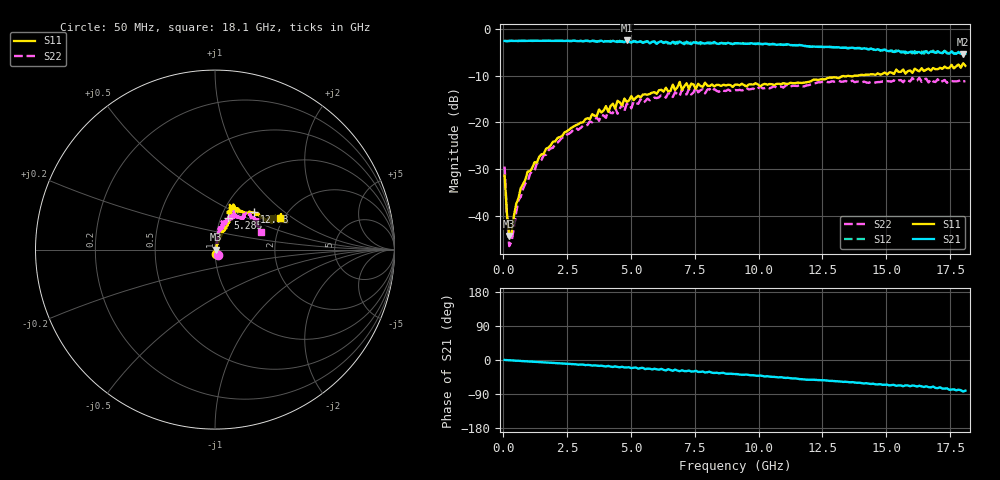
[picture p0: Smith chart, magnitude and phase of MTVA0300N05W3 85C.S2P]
! Network Analyzer HP8720D.06.14 Serial No. US36140669
!  7 Jul 2005  09:27:54
! Frequency  S11  S21  S12  S22
# HZ  S  DB R 50
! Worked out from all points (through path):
!   201 points, 50 MHz to 18.1 GHz, reference 50 ohm
!   highest |S21| = -2.42 dB at 4.833 GHz (marker M1); lowest = -5.3 dB at 18.01 GHz (marker M2)
!   group delay of S21, straight-line fit = 12.3 ps
!   lowest |S11| = -44.4 dB at 230.5 MHz (marker M3), VSWR 1.01, Z = 50.6 - j0.127 ohm
!   |S11| at or under -10 dB: start of sweep to 13.74 GHz; 13.83626 GHz to 13.87192 GHz (35.66 MHz wide, 0.257 % of centre)
!   |S22| runs from -46.6 to -10.4 dB; largest |S21 - S12| = 0.045
!   S11 on the Smith chart (normalised r, x): 50 MHz: 1.02, -0.05; 5.285 GHz: 1.08, +0.40; 12.78 GHz: 1.39, +0.64; 18.1 GHz: 1.93, +0.80
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5e7  -31.42 -72.1  -2.52 0.1  -2.51 0.2  -29.48 -61.3
1.4025e8  -39.49 -54.7  -2.56 -0.4  -2.56 -0.4  -39.91 -62.7
2.305e8  -44.39 -12.0  -2.53 -0.7  -2.52 -0.8  -46.57 -31.9
3.2075e8  -43.78 33.0  -2.50 -0.9  -2.52 -1.0  -45.61 32.0
5.915e8  -36.28 63.3  -2.52 -2.0  -2.54 -2.1  -36.69 71.9
1.04275e9  -30.49 70.9  -2.48 -4.0  -2.50 -4.0  -31.09 73.4
1.94525e9  -24.15 68.6  -2.51 -7.8  -2.51 -7.7  -25.44 77.1
3.1185e9  -20.01 67.6  -2.58 -12.0  -2.60 -12.5  -20.72 78.9
4.83325e9  -15.60 71.0  -2.42 -19.5  -2.69 -20.3  -16.07 67.5
5.2845e9  -14.29 67.8  -2.76 -23.0  -2.83 -22.2  -16.04 67.0
6.09675e9  -13.11 65.0  -2.77 -25.6  -2.66 -25.2  -14.62 66.7
6.7285e9  -13.08 71.6  -2.85 -25.4  -3.17 -26.5  -13.53 60.8
6.909e9  -11.32 67.8  -2.65 -29.6  -2.77 -27.4  -14.32 61.1
6.99925e9  -13.02 67.7  -2.97 -27.3  -3.15 -29.8  -12.92 61.4
7.17975e9  -11.61 71.8  -2.69 -29.3  -3.02 -27.6  -14.01 57.6
7.54075e9  -12.81 64.4  -2.94 -28.5  -2.79 -31.9  -12.44 64.1
9.075e9  -11.89 64.2  -3.03 -37.0  -2.99 -37.1  -13.06 54.8
1.21435e10  -10.85 47.7  -3.72 -52.1  -3.66 -52.1  -11.69 50.2
1.277525e10  -10.38 43.4  -3.80 -55.1  -3.82 -54.7  -11.38 45.7
1.512175e10  -9.26 27.1  -4.72 -67.1  -4.45 -66.6  -11.21 39.5
1.800975e10  -7.32 20.6  -5.32 -83.3  -5.03 -83.2  -11.26 25.4
1.81e10  -7.87 25.5  -5.24 -80.9  -5.54 -80.8  -11.13 21.2
